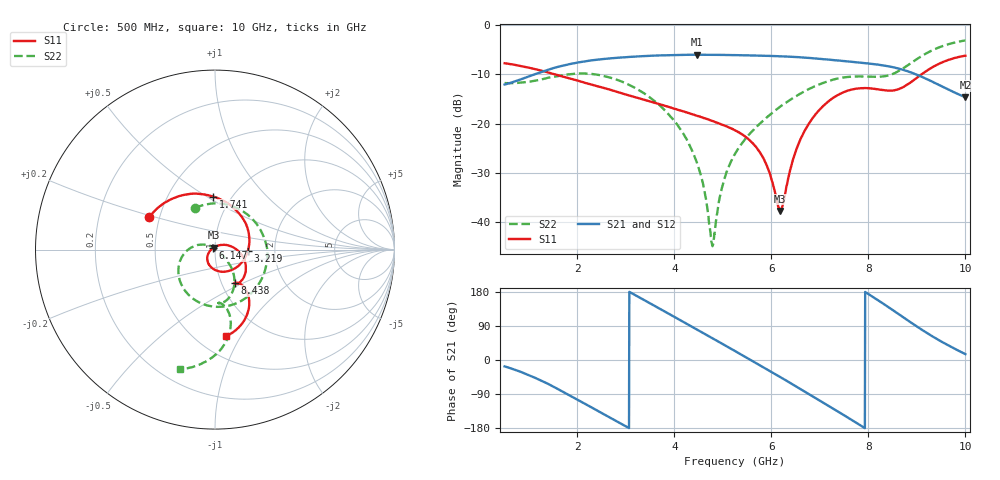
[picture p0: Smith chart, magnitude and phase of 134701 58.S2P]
!  2-Port S-parameters saved by WinCal
! VAR MeasName=S-Parameters (CALIBRATED_DATA) read from VNA (N5242A)
! VAR MeasDate=2013-7-3 16:40:51
! VAR NAME=134701 58
! VAR FILENAME=134701 58.S2P
! VAR DATE=2013-7-3 16:40:51
! VAR PHYS_PORTS=1,2
# Hz S MA R 50
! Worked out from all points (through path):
!   1601 points, 500 MHz to 10 GHz, reference 50 ohm
!   highest |S21| = -6.05 dB at 4.46 GHz (marker M1); lowest = -14.7 dB at 10 GHz (marker M2)
!   lowest |S11| = -37.7 dB at 6.182 GHz (marker M3), VSWR 1.03, Z = 49.3 + j1.09 ohm
!   |S11| at or under -10 dB: 1.527 GHz to 9.1 GHz (7.573 GHz wide, 143 % of centre)
!   |S22| runs from -44.8 to -3.2 dB; largest |S21 - S12| = 0.0016
!   S11 on the Smith chart (normalised r, x): 500 MHz: 0.44, +0.19; 1.741 GHz: 0.82, +0.53; 3.219 GHz: 1.45, -0.02; 6.147 GHz: 0.98, +0.02; 8.438 GHz: 1.15, -0.45; 10 GHz: 0.68, -0.87
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5e8  0.4086 154.0  0.2487 -16.9  0.248 -16.8  0.257 115.6
1.224375e9  0.3469 117.8  0.328 -52.7  0.3281 -52.6  0.2773 20.9
1.740938e9  0.2954 91.9  0.39 -86.4  0.3904 -86.4  0.3108 -38.9
2.085312e9  0.2657 73.2  0.4219 -110.4  0.4219 -110.4  0.3221 -72.6
2.702812e9  0.2184 34.6  0.4586 -154.2  0.4582 -154.2  0.2897 -121.7
3.219375e9  0.1833 -2.3  0.4779 169.4  0.4779 169.4  0.2253 -154.2
3.670625e9  0.1586 -35.2  0.4902 137.3  0.4894 137.3  0.1571 -177.7
4.460312e9  0.1205 -82.3  0.4981 80.7  0.4985 80.7  0.04062 145.6
4.602812e9  0.1139 -89.0  0.4975 70.5  0.498 70.4  0.02295 135.2
4.786875e9  0.1063 -96.9  0.4972 57.2  0.4974 57.2  0.005752 55.0
4.994688e9  0.09726 -105.1  0.4956 42.2  0.496 42.2  0.02359 -23.3
5.25e9  0.08562 -115.5  0.4933 23.7  0.4935 23.6  0.04948 -35.1
5.802188e9  0.04781 -145.4  0.487 -16.6  0.4871 -16.7  0.1043 -44.2
6.146562e9  0.01427 144.5  0.4806 -42.3  0.481 -42.3  0.1441 -48.9
6.182188e9  0.01305 122.1  0.4801 -45.0  0.4799 -45.0  0.1488 -49.4
6.502812e9  0.05258 30.7  0.4718 -69.2  0.4724 -69.3  0.1889 -55.5
6.835312e9  0.1108 4.0  0.4599 -94.8  0.4603 -94.8  0.231 -62.9
7.6725e9  0.222 -43.5  0.4209 -159.5  0.4217 -159.6  0.2992 -82.7
8.420625e9  0.2157 -59.8  0.3796 138.7  0.3796 138.7  0.3081 -82.1
8.438438e9  0.2156 -59.6  0.3775 137.2  0.3782 137.2  0.3104 -81.7
9.26375e9  0.358 -57.8  0.2734 66.9  0.2741 66.8  0.536 -84.8
1e10  0.4867 -82.9  0.1851 15.5  0.1854 15.4  0.6943 -106.4
